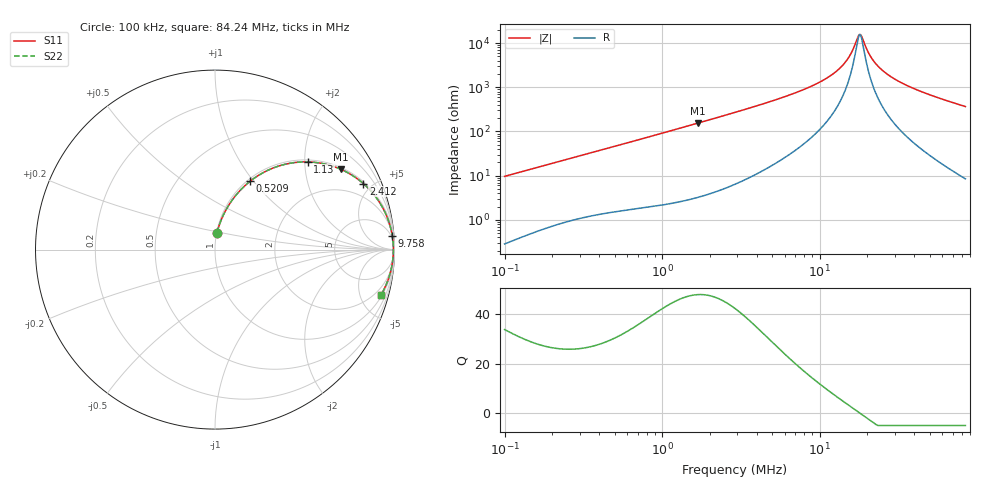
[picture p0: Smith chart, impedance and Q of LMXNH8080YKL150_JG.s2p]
! LMXNH8080YKL150_JG  S-PARAMETER MODEL  ( General Type )
! Model Generated by TAIYO YUDEN Corporation (https://www.yuden.co.jp/en/)
! Version 1.0
! TAIYO YUDEN Control No. 191025NI43SB-FBB
! Copyright(c) 2019 TAIYO YUDEN CO.,LTD. All Rights Reserved.
! Product Description (link to TY-COMPAS)
! https://ds.yuden.co.jp/TYCOMPAS/or/detail?pn=LMXNH8080YKL150MJG&u=M
! Products Name : Inductors
! Characteristics :
!  Inductance : 15 uH , SRF(min) : 16 MHz , DC Resistance(max) : 0.065 Ohm
!  Rated Current : Saturation :2900 mA , Temp Rise : 2400 mA (40 degC)
!  Case Size : 8.0 x 8.0 / 0.315 x 0.315 [mm/inch] , Thickness : 4 / 0.157 [mm/inch]
!  (Conditions: Temperature = 25 degC , DC Bias Current/Voltage = 0A / 0V)
! External Node Assignments :
!  1  o---GGG---o  2
! GND o---------o GND
! Frequency Range : 0.1MHz  -  84.23641MHz  [ 402 STEP ]
# MHz S RI R 50
! Freq[MHz].  S11 Real  S11 Imag  S21 Real  S21 Imag  S12 Real  S12 Imag  S22 Real  S22 Imag
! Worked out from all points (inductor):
!   401 points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, 100 kHz to 84.24 MHz, reference 50 ohm
!   read as one part in series: L = 15.3 uH near 103.4 kHz
!   highest Q = 47.9 at 1.693 MHz (marker M1), where L = 14.6 uH
!   self-resonance near 17.89 MHz
!   S11 on the Smith chart (normalised r, x): 100 kHz: 1.01, +0.19; 520.9 kHz: 1.03, +0.96; 1.13 MHz: 1.05, +2.07; 2.412 MHz: 1.10, +4.46; 9.758 MHz: 3, +25; 84.24 MHz: 1.17, -7.33
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0.1  0.012 0.095  0.988 -0.095  0.988 -0.095  0.012 0.095
0.309045  0.0854 0.2611  0.9146 -0.2611  0.9146 -0.2611  0.0854 0.2611
0.520892  0.1948 0.3802  0.8052 -0.3802  0.8052 -0.3802  0.1948 0.3802
0.955086  0.4342 0.4837  0.5658 -0.4837  0.5658 -0.4837  0.4342 0.4837
1.130264  0.5159 0.4886  0.4841 -0.4886  0.4841 -0.4886  0.5159 0.4886
1.693207  0.7028 0.4467  0.2972 -0.4467  0.2972 -0.4467  0.7028 0.4467
2.411563  0.8271 0.3674  0.1729 -0.3674  0.1729 -0.3674  0.8271 0.3674
2.902351  0.8739 0.3203  0.1261 -0.3203  0.1261 -0.3203  0.8739 0.3203
5.597398  0.9631 0.1702  0.0369 -0.1702  0.0369 -0.1702  0.9631 0.1702
8.96956  0.9852 0.0905  0.0148 -0.0905  0.0148 -0.0905  0.9852 0.0905
9.75753  0.9874 0.0783  0.0126 -0.0783  0.0126 -0.0783  0.9874 0.0783
12.14559  0.9912 0.0488  0.00875 -0.0488  0.00875 -0.0488  0.9912 0.0488
14.13326  0.9928 0.0296  0.0072 -0.0296  0.0072 -0.0296  0.9928 0.0296
15.63597  0.9934 0.0172  0.00659 -0.0172  0.00659 -0.0172  0.9934 0.0172
17.29846  0.9937 0.00497  0.0063 -0.00497  0.0063 -0.00497  0.9937 0.00497
17.89101  0.9937 0.000899  0.00628 -0.000899  0.00628 -0.000899  0.9937 0.000899
18.50386  0.9937 -0.00317  0.00628 0.00317  0.00628 0.00317  0.9937 -0.00317
20.47127  0.9935 -0.0154  0.0065 0.0154  0.0065 0.0154  0.9935 -0.0154
22.26966  0.9931 -0.0257  0.00692 0.0257  0.00692 0.0257  0.9931 -0.0257
27.71995  0.9909 -0.0535  0.00912 0.0535  0.00912 0.0535  0.9909 -0.0535
42.94868  0.9798 -0.1169  0.0202 0.1169  0.0202 0.1169  0.9798 -0.1169
84.23641  0.9258 -0.2509  0.0742 0.2509  0.0742 0.2509  0.9258 -0.2509
